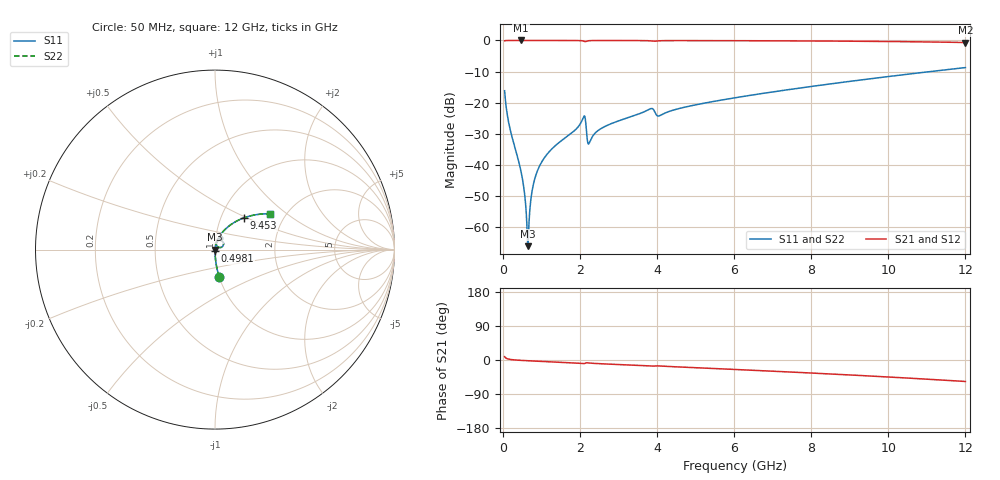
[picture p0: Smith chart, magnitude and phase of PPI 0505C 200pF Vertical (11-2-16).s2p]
# GHz S MA R 50
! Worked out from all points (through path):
!   1601 points, 50 MHz to 12 GHz, reference 50 ohm
!   highest |S21| = 0.00 dB at 475.7 MHz (marker M1); lowest = -0.7 dB at 12 GHz (marker M2)
!   group delay of S21, straight-line fit = 13.1 ps
!   lowest |S11| = -66.0 dB at 655 MHz (marker M3), VSWR 1.00, Z = 50 + j0.00401 ohm
!   |S11| at or under -10 dB: start of sweep to 11.08 GHz
!   |S22| runs from -66.0 to -8.7 dB; largest |S21 - S12| = 0
!   S11 on the Smith chart (normalised r, x): 50 MHz: 1.00, -0.32; 498.1 MHz: 1.00, -0.01; 9.453 GHz: 1.28, +0.48; 12 GHz: 1.67, +0.77
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0.05  0.1561 -81.1  0.9875 8.8  0.9875 8.8  0.1561 -81.1
0.1844375  0.03965 -87.8  0.9989 1.7  0.9989 1.7  0.03965 -87.8
0.4757188  0.007894 -87.8  0.9995 -1.0  0.9995 -1.0  0.007894 -87.8
0.498125  0.006726 -87.3  0.9995 -1.1  0.9995 -1.1  0.006726 -87.3
0.557875  0.003911 -84.6  0.9995 -1.5  0.9995 -1.5  0.003911 -84.6
0.617625  0.001464 -72.4  0.9995 -1.8  0.9995 -1.8  0.001464 -72.4
0.6549687  0.0005011 4.6  0.9995 -2.0  0.9995 -2.0  0.0005011 4.6
0.6923125  0.001507 68.1  0.9994 -2.2  0.9994 -2.2  0.001507 68.1
0.7520625  0.003506 78.9  0.9994 -2.5  0.9994 -2.5  0.003506 78.9
0.8043438  0.005181 81.3  0.9994 -2.7  0.9994 -2.7  0.005181 81.3
0.9835938  0.01044 83.2  0.9993 -3.6  0.9993 -3.6  0.01044 83.2
2.044156  0.04999 72.0  0.9909 -9.0  0.9909 -9.0  0.04999 72.0
2.111375  0.06138 52.3  0.9694 -9.5  0.9694 -9.5  0.06138 52.3
2.253281  0.02318 61.8  0.9916 -8.1  0.9916 -8.1  0.02318 61.8
2.611781  0.04051 77.6  0.9974 -10.2  0.9974 -10.2  0.04051 77.6
3.806781  0.07904 67.1  0.9872 -16.0  0.9872 -16.0  0.07904 67.1
4.038312  0.06136 62.0  0.9848 -15.6  0.9848 -15.6  0.06136 62.0
6.025  0.1204 64.3  0.9908 -25.0  0.9908 -25.0  0.1204 64.3
8.019156  0.1833 55.0  0.9807 -34.4  0.9807 -34.4  0.1833 55.0
9.453156  0.2393 47.7  0.9682 -41.8  0.9682 -41.8  0.2393 47.7
10.01331  0.2641 44.6  0.9616 -44.9  0.9616 -44.9  0.2641 44.6
12  0.3669 32.9  0.9267 -56.7  0.9267 -56.7  0.3669 32.9
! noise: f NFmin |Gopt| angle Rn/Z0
0.05  0.0003251  0.8399  0.2898  0.00043
1.372  0.003207  0.6104  4.006  0.001524
2.701  0.006364  0.6135  7.86  0.003045
4.031  0.02383  0.8262  12.08  0.02852
5.36  0.009572  0.5229  14.81  0.003465
6.682  0.01097  0.4943  17.88  0.003652
8.012  0.01276  0.4862  20.93  0.004126
9.341  0.01479  0.4878  23.9  0.004758
10.67  0.01708  0.4968  26.83  0.005569
12  0.01972  0.5122  29.75  0.006622
